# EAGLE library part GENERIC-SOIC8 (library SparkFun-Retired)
A placeholder for generic narrow & wide SOIC8 foorptints - used on the DIP adapter board. Has strange reference to IC-10141, a Seven Band Graphic Equalizer Display Filter SOIC-8 VFP: IC-10141
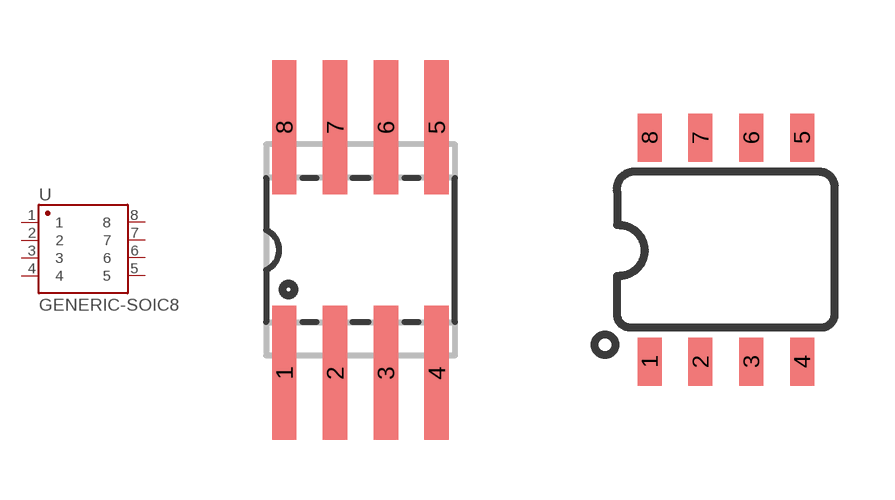
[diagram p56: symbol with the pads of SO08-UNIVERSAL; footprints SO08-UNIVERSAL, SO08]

Designator prefix U

## GENERIC-SOIC8  [SO08-UNIVERSAL]
1  1
2  2
3  3
4  4
5  5
6  6
7  7
8  8

## GENERIC-SOIC8MSGEQ7N-FILTER (PROD_ID: IC-10141)  [SO08]
Pads as for SO08-UNIVERSAL

## Footprint SO08-UNIVERSAL (pad centres in mm)
SOIC-08 footprint wth long lands. To fit both narrow and wide SOICs - for SOIC-to-DIP adapter board. Not recommended if you're trying to fit a specific chip.
smd 0.61 x 3.353: 1 -1.905,-3.073; 2 -0.635,-3.073; 3 0.635,-3.073; 4 1.905,-3.073; 5 1.905,3.073; 6 0.635,3.073; 7 -0.635,3.073; 8 -1.905,3.073

## Footprint SO08 (pad centres in mm)
SOIC, 0.15 inch width
smd 0.6 x 1.2: 1 -1.905,-2.8; 2 -0.635,-2.8; 3 0.635,-2.8; 4 1.905,-2.8; 5 1.905,2.8; 6 0.635,2.8; 7 -0.635,2.8; 8 -1.905,2.8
